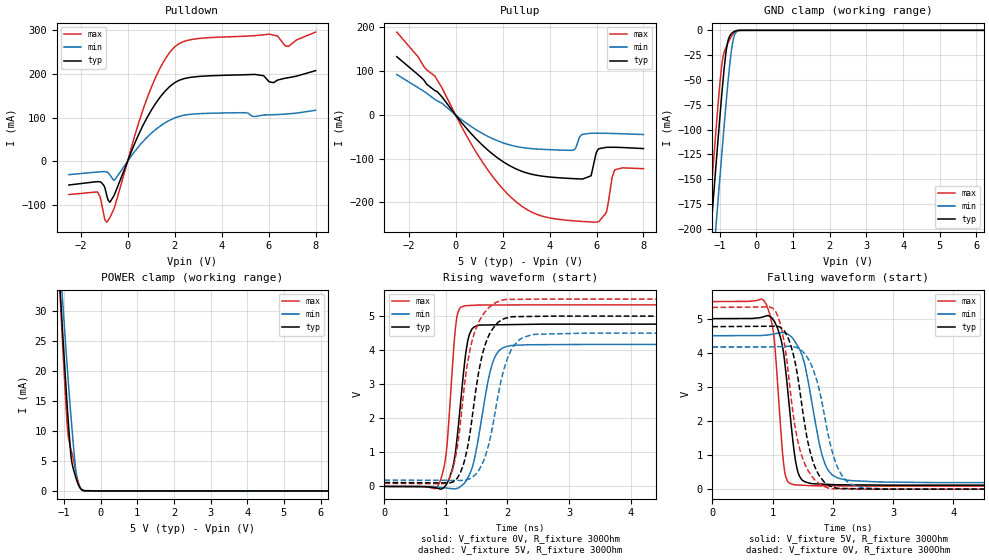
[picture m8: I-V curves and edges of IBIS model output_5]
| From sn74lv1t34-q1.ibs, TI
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[Model]   output_5
Model_type   Output
Polarity   Non-Inverting
Vmeas = 1.5
Vref = 0.9
Cref = 15pF
Rref = 100000
|   typ   min   max
C_comp   4.947pF   4.835pF   5.043pF
[Voltage Range]   5   4.5   5.5
[Temperature Range]   27   125   -40
[Pullup Reference]   5   4.5   5.5
[Pulldown Reference]   -0   0   0
[Power Clamp Reference]   5   4.5   5.5
[GND Clamp Reference]   0   0   0
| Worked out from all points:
|   slope of the pulldown table from 0 to 0.75 V, typ, clamps not added: 8.16 ohm
|   slope of the pullup table from 0 to 0.75 V, typ, clamps not added: 15.7 ohm
|   GND clamp passes 1 mA (typ) near -0.59 V on its own axis
|   POWER clamp passes 1 mA (typ) near -0.60 V on its own axis
|   falling waveform, V_fixture 5V, R_fixture 300Ohm: 20-80 % time 179ps typ, 278ps min, 134ps max; typ from 5 V to 0.116 V
|   rising waveform, V_fixture 0V, R_fixture 300Ohm: 20-80 % time 164ps typ, 247ps min, 125ps max; typ from 0 V to 4.76 V
|   rising waveform, V_fixture 5V, R_fixture 300Ohm: 20-80 % time 271ps typ, 311ps min, 262ps max; typ from 0.116 V to 5 V
|   falling waveform, V_fixture 0V, R_fixture 300Ohm: 20-80 % time 284ps typ, 331ps min, 272ps max; typ from 4.76 V to 0 V
[Pulldown]
|   Voltage   I(typ)   I(min)   I(max)
-2.5V     -54.17mA   -30.47mA   -76mA
-1.292V   -46.43mA   -24.52mA   -69.97mA
-998.5mV  -56.07mA   -23.49mA   -125.9mA
-872.5mV  -81.07mA   -24.92mA   -138.7mA
-757mV    -93.39mA   -30.82mA   -128.9mA
-547mV    -74.32mA   -42.13mA   -103.1mA
1.018V    117.6mA    64.62mA    170mA
2.162V    184.3mA    102.1mA    268mA
5.407V    198.7mA    102.2mA    287.3mA
6.026V    181.7mA    106.1mA    290.8mA
6.845V    191.1mA    108.5mA    262.7mA
8V        207.3mA    116.6mA    295.4mA
[GND Clamp]
|   Voltage   I(typ)   I(min)   I(max)
-2.5V     -817.8mA   -872.3mA   -789.1mA
-1.303V   -231.2mA   -292.1mA   -196.1mA
-1.23V    -196.2mA   -257.3mA   -160.8mA
-1.125V   -146.7mA   -208.1mA   -111.2mA
-1.062V   -117.5mA   -178.9mA   -82.22mA
-946mV    -65.86mA   -126.2mA   -35.86mA
-830.5mV  -22.76mA   -75.49mA   -17.36mA
-767.5mV  -9.785mA   -49.8mA    -12.22mA
-694mV    -3.965mA   -24.23mA   -6.893mA
-589mV    -891.1uA   -3.999mA   -1.764mA
-431.5mV  -12.85uA   -82.5uA    -10.98uA
8V        0A         0A         0A
[Pullup]
|   Voltage   I(typ)   I(min)   I(max)
-2.5V     133.2mA    92.38mA    189.5mA
-872.5mV  55.54mA    35.32mA    88.38mA
1.532V    -87.54mA   -53.13mA   -137.5mA
3.149V    -134.5mA   -76.7mA    -219.8mA
5.018V    -145.8mA   -80.62mA   -242.3mA
5.407V    -146.7mA   -44.46mA   -243.8mA
5.763V    -139.4mA   -41.98mA   -244.9mA
6.058V    -79.55mA   -41.85mA   -244.8mA
6.415V    -74.24mA   -42.14mA   -223.5mA
6.667V    -74mA      -42.47mA   -142.1mA
6.771V    -74.07mA   -42.63mA   -126.1mA
8V        -77.02mA   -44.9mA    -123mA
[POWER Clamp]
|   Voltage   I(typ)   I(min)   I(max)
-2.5V     147.9mA    120.2mA    180.7mA
-1.177V   41.53mA    40.53mA    41.66mA
-1.072V   30.45mA    34.72mA    28.9mA
-1.04V    27.19mA    32.3mA     25.19mA
-946mV    17.75mA    23.94mA    14.69mA
-893.5mV  12.85mA    19.46mA    9.879mA
-799mV    5.488mA    11.92mA    6.762mA
-725.5mV  3.307mA    6.625mA    4.806mA
-652mV    1.818mA    2.364mA    2.632mA
-589mV    837.6uA    921.4uA    1.128mA
-494.5mV  114.2uA    194.6uA    87.23uA
8V        0A         0A         0A
[Ramp]
R_load = 300
|   typ   min   max
dV/dt_r   2.85909/1.64227e-10   2.50123/2.46513e-10   3.1981/1.25452e-10
dV/dt_f   2.93049/1.78709e-10   2.58732/2.77607e-10   3.24613/1.34209e-10
[Falling Waveform]
V_fixture = 5V
V_fixture_min = 4.5V
V_fixture_max = 5.5V
R_fixture = 300Ohm
C_fixture = 0F
|   Time   V(typ)   V(min)   V(max)
0s        5V         4.5V       5.5V
899.3ps   5.081V     4.518V     5.399V
1.027ns   4.927V     4.552V     4.401V
1.158ns   4.241V     4.593V     1.212V
1.221ns   3.406V     4.569V     344.8mV
1.351ns   1.197V     4.381V     132.3mV
1.482ns   281.8mV    3.954V     115.5mV
1.867ns   144.1mV    750.4mV    97.94mV
2.206ns   127.4mV    272.9mV    94.17mV
15ns      115.8mV    187.8mV    89.78mV
[Rising Waveform]
V_fixture = 0V
V_fixture_min = 0V
V_fixture_max = 0V
R_fixture = 300Ohm
C_fixture = 0F
|   Time   V(typ)   V(min)   V(max)
0s        1.427uV    1.371uV    1.299uV
889.8ps   -68.08mV   -22.9mV    87.87mV
1.008ns   60.88mV    -47.63mV   1.036V
1.131ns   733mV      -73.02mV   4.163V
1.196ns   1.681V     -48.48mV   5.116V
1.304ns   3.643V     105mV      5.301V
1.426ns   4.628V     553.3mV    5.315V
1.754ns   4.742V     3.607V     5.325V
2.032ns   4.749V     4.128V     5.327V
15ns      4.765V     4.169V     5.33V
[Rising Waveform]
V_fixture = 5V
V_fixture_min = 4.5V
V_fixture_max = 5.5V
R_fixture = 300Ohm
C_fixture = 0F
|   Time   V(typ)   V(min)   V(max)
0s        115.8mV    187.8mV    89.78mV
995.3ps   103mV      178.1mV    107.5mV
1.184ns   245.3mV    176.3mV    1.154V
1.339ns   1.054V     197.9mV    3.493V
1.456ns   2.432V     311.6mV    4.468V
1.646ns   4.203V     924.2mV    5.145V
1.926ns   4.908V     3.332V     5.475V
2.163ns   4.985V     4.258V     5.493V
2.456ns   4.992V     4.466V     5.498V
15ns      5V         4.5V       5.5V
[Falling Waveform]
|Gnd
V_fixture = 0V
V_fixture_min = 0V
V_fixture_max = 0V
R_fixture = 300Ohm
C_fixture = 0F
|   Time   V(typ)   V(min)   V(max)
0s        4.765V     4.169V     5.33V
1.043ns   4.78V      4.174V     5.225V
1.186ns   4.655V     4.184V     4.369V
1.288ns   4.292V     4.191V     2.977V
1.481ns   2.51V      4.059V     989.1mV
1.671ns   798mV      3.519V     330.4mV
1.926ns   115.5mV    1.563V     29.66mV
2.163ns   20.64mV    368.4mV    9.044mV
2.571ns   7.108mV    32.68mV    429.2uV
15ns      1.427uV    1.371uV    1.299uV
